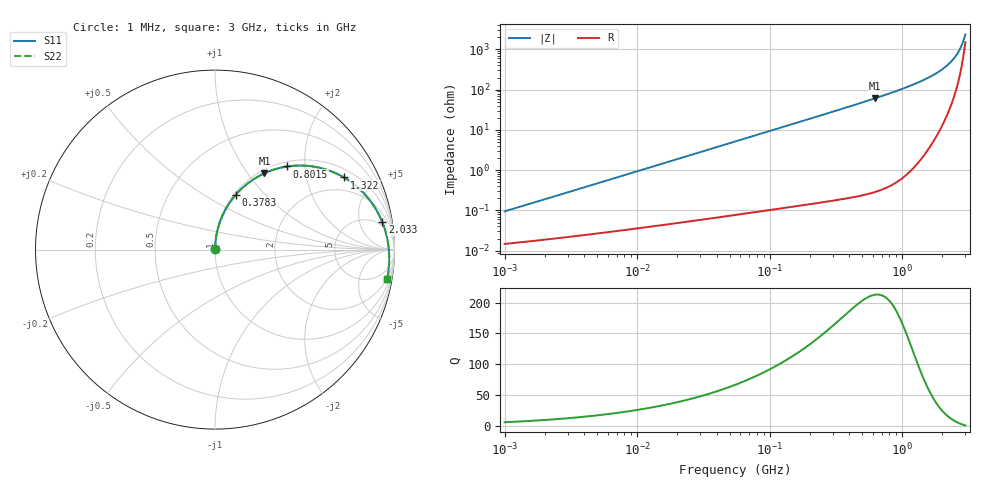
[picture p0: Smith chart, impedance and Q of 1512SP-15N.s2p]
# MHz  S  MA  R  50
!Freq  MagS11  AngS11  MagS21  AngS21  MagS12  AngS12  MagS22  AngS22
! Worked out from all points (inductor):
!   801 points, 1 MHz to 3 GHz, reference 50 ohm
!   read as one part in series: L = 14.9 nH near 1.041 MHz
!   highest Q = 213 at 624.1 MHz (marker M1), where L = 15.5 nH
!   S11 on the Smith chart (normalised r, x): 1 MHz: 1.00, +0.00; 378.3 MHz: 1.02, +0.70; 801.5 MHz: 1.09, +1.62; 1.322 GHz: 1.34, +3.34; 2.033 GHz: 4, +11; 3 GHz: 2, -11
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1  0.0009167 80.7  0.9999 -0.1  0.9999 -0.1  0.0009167 80.7
3.824029  0.003468 85.8  0.9998 -0.2  0.9998 -0.2  0.003468 85.8
14.47755  0.0131 87.4  0.9995 -0.8  0.9995 -0.8  0.0131 87.4
54.81117  0.04953 86.1  0.998 -3.0  0.998 -3.0  0.04952 86.1
113.8185  0.1025 83.1  0.9937 -6.3  0.9937 -6.3  0.1025 83.1
209.5995  0.187 78.0  0.9809 -11.5  0.9809 -11.5  0.1869 78.0
288.7352  0.2546 73.9  0.9654 -15.8  0.9654 -15.8  0.2545 73.9
378.3323  0.3279 69.2  0.9428 -20.5  0.9428 -20.5  0.3279 69.2
490.7947  0.4142 63.5  0.9081 -26.2  0.9081 -26.2  0.4141 63.5
624.0682  0.5069 57.0  0.8596 -32.7  0.8596 -32.7  0.5067 57.0
793.5315  0.609 49.4  0.7902 -40.3  0.7902 -40.3  0.6088 49.4
801.5144  0.6133 49.0  0.7868 -40.7  0.7868 -40.7  0.6131 49.0
1039.771  0.7267 39.3  0.6823 -50.3  0.6823 -50.3  0.7265 39.3
1322.117  0.8233 29.2  0.5592 -60.2  0.5592 -60.2  0.823 29.2
1681.133  0.9014 18.4  0.4145 -70.4  0.4145 -70.4  0.9011 18.4
2033.286  0.9446 9.4  0.2901 -78.2  0.2901 -78.2  0.9443 9.3
2292.791  0.962 3.5  0.2098 -82.1  0.2098 -82.1  0.9618 3.5
2534.173  0.9705 -1.4  0.1433 -83.6  0.1433 -83.6  0.9704 -1.4
2718.106  0.9732 -4.9  0.098 -81.8  0.098 -81.8  0.9732 -4.9
2800.967  0.9736 -6.4  0.0793 -79.2  0.0793 -79.2  0.9737 -6.4
2915.39  0.9734 -8.4  0.05578 -71.5  0.05578 -71.5  0.9735 -8.4
3000  0.9728 -9.8  0.04113 -59.6  0.04113 -59.6  0.9729 -9.8
